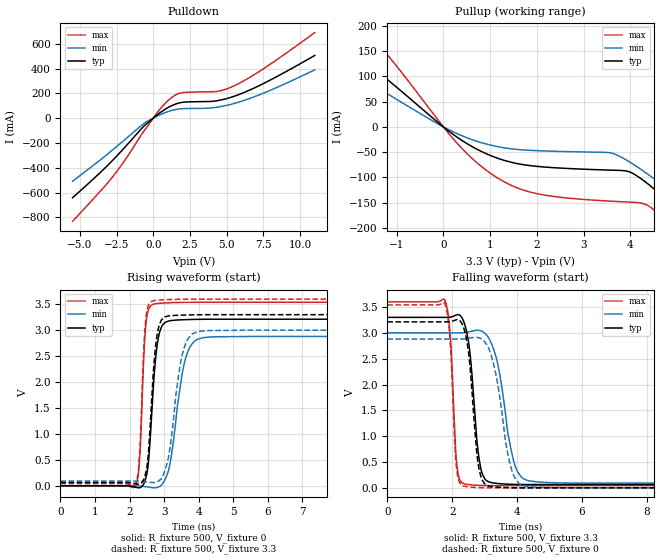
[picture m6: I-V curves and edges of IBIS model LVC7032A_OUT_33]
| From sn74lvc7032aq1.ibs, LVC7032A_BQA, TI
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[Model]   LVC7032A_OUT_33
Model_type  Output
Vref =   0
Rref =   500
Cref =   50p
Vmeas =   1.5
| variable   typ   min   max
C_comp   6.12pF   3.46pF   8.37pF
| C_pullup   5.73pF   3.46pF   7.15pF
| C_pulldown   6.51pF   4.19pF   8.37pF
[Temperature Range]   40   100   -40
| Ambient temperature   25   85   -40
[Voltage range]   3.3   3   3.6
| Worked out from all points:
|   slope of the pulldown table from 0 to 0.495 V, typ, clamps not added: 10.7 ohm
|   slope of the pullup table from 0 to 0.495 V, typ, clamps not added: 15.2 ohm
|   rising waveform, R_fixture 500, V_fixture 0: 20-80 % time 203ps typ, 358ps min, 132ps max; typ from 0 V to 3.21 V
|   falling waveform, R_fixture 500, V_fixture 3.3: 20-80 % time 257ps typ, 441ps min, 158ps max; typ from 3.3 V to 0.065 V
|   rising waveform, R_fixture 500, V_fixture 3.3: 20-80 % time 193ps typ, 334ps min, 130ps max; typ from 0.065 V to 3.3 V
|   falling waveform, R_fixture 500, V_fixture 0: 20-80 % time 250ps typ, 434ps min, 157ps max; typ from 3.21 V to 0 V
[Pulldown]
| LVC7032A_OUT_33
|   Voltage   I(typ)   I(min)   I(max)
-5.5V     -642.1mA   -509.2mA   -832.1mA
-3.645V   -442.6mA   -340.3mA   -594.1mA
-2.71V    -333.2mA   -250.5mA   -464.6mA
-1.885V   -228.4mA   -168.1mA   -330.7mA
-620mV    -62.4mA    -41.49mA   -102.1mA
455mV     42.83mA    26.93mA    71.74mA
1.215V    98.07mA    60.46mA    162.3mA
1.91V     125.9mA    75.23mA    203.5mA
4.31V     139.6mA    87.57mA    214.6mA
5.45V     173.8mA    116.3mA    257.3mA
7.53V     280.4mA    202.4mA    399.9mA
11V       505.3mA    389mA      689.8mA
[Pullup]
| LVC7032A_OUT_33
|   Voltage   I(typ)   I(min)   I(max)
-5.5V     404.4mA    310.8mA    569.2mA
-3.515V   265mA      197.3mA    383.4mA
-2.48V    190.1mA    138.3mA    280.1mA
-1.635V   127.1mA    90.28mA    191.1mA
505mV     -33.05mA   -21.44mA   -52.79mA
1.855V    -76.61mA   -46.34mA   -128.9mA
3.7V      -85.85mA   -55.1mA    -147.6mA
4.24V     -103.3mA   -84.95mA   -151mA
4.895V    -154.7mA   -130.6mA   -201.2mA
5.365V    -197.4mA   -166.8mA   -253mA
5.825V    -241.6mA   -203.9mA   -307.6mA
11V       -786.6mA   -661.2mA   -974mA
[Ramp]
| LVC7032A_OUT_33
| variable   typ   min   max
dV/dt_r   1.95/2.10E-10   1.75/3.93E-10   2.15/1.36E-10
dV/dt_f   1.97/2.73E-10   1.77/4.60E-10   2.17/1.66E-10
R_load = 500
[Rising Waveform]
| LVC7032A_OUT_33
R_fixture =   500
C_fixture =   0
L_fixture =   0
V_fixture =   0
V_fixture_min = 0
V_fixture_max = 0
|   Time   V(typ)   V(min)   V(max)
0s        184.9pV    3.596nV    20.95pV
2.18ns    -26.84mV   1.09mV     7.124mV
2.3ns     -34.96mV   -3.206mV   614.2mV
2.48ns    176.5mV    -17.86mV   3.158V
2.75ns    2.432V     -37.75mV   3.511V
2.885ns   2.996V     -5.668mV   3.521V
3.13ns    3.177V     299mV      3.53V
3.64ns    3.205V     2.497V     3.538V
4.125ns   3.211V     2.858V     3.539V
24.99ns   3.212V     2.88V      3.539V
[Falling Waveform]
| LVC7032A_OUT_33
R_fixture =   500
C_fixture =   0
L_fixture =   0
V_fixture =   3.3
V_fixture_min = 3
V_fixture_max = 3.6
|   Time   V(typ)   V(min)   V(max)
0s        3.3V       3V         3.6V
1.785ns   3.3V       3V         3.618V
1.955ns   3.305V     2.999V     2.831V
2.145ns   3.351V     2.999V     447.9mV
2.385ns   3.168V     3.004V     74.71mV
2.845ns   507.6mV    3.046V     47.32mV
3.225ns   98.77mV    2.773V     43mV
3.89ns    66.77mV    532.9mV    41.9mV
4.37ns    63.65mV    134.7mV    41.89mV
24.99ns   64.52mV    92.1mV     41.93mV
[Rising Waveform]
| LVC7032A_OUT_33
R_fixture =   500
C_fixture =   0
L_fixture =   0
V_fixture =   3.3
V_fixture_min = 3
V_fixture_max = 3.6
|   Time   V(typ)   V(min)   V(max)
0s        64.52mV    92.1mV     41.93mV
2.18ns    40.01mV    92.93mV    56.54mV
2.29ns    35.04mV    89.23mV    623.5mV
2.465ns   243.2mV    76.95mV    3.184V
2.69ns    2.211V     64.1mV     3.57V
2.935ns   3.207V     153.4mV    3.586V
3.14ns    3.278V     606.3mV    3.592V
3.535ns   3.292V     2.554V     3.598V
4.005ns   3.298V     2.979V     3.6V
24.99ns   3.3V       3V         3.6V
[Falling Waveform]
| LVC7032A_OUT_33
R_fixture =   500
C_fixture =   0
L_fixture =   0
V_fixture =   0
V_fixture_min = 0
V_fixture_max = 0
|   Time   V(typ)   V(min)   V(max)
0s        3.212V     2.88V      3.539V
1.78ns    3.212V     2.879V     3.555V
1.935ns   3.216V     2.879V     2.852V
2.13ns    3.253V     2.879V     412.2mV
2.355ns   3.098V     2.882V     32.78mV
2.81ns    434.4mV    2.907V     5.334mV
3.135ns   33.08mV    2.693V     1.347mV
3.815ns   2.294mV    393.7mV    -8.404uV
4.32ns    -635.7uV   19.03mV    -35.02uV
24.99ns   -530.1pV   20.42nV    18.32nV
